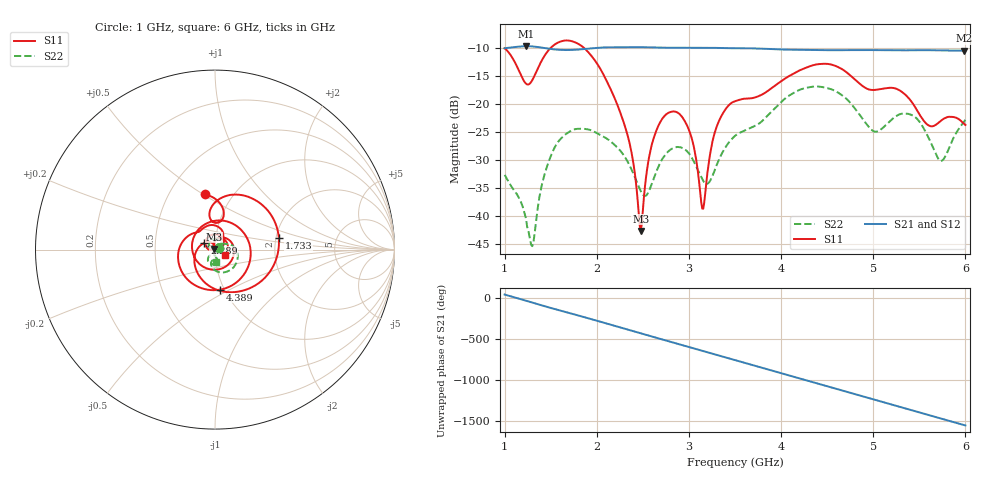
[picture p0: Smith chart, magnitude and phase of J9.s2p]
!Agilent Technologies,E8364B,MY43040528,A.07.50.67
!Agilent E8364B: A.07.50.67
!Date: Sunday, March 01, 2026 19:10:28
!Correction: S11(Full 2 Port(1,2))
!S21(Full 2 Port(1,2))
!S12(Full 2 Port(1,2))
!S22(Full 2 Port(1,2))
!S2P File: Measurements: S11, S21, S12, S22:
# Hz S  dB  R 50
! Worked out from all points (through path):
!   451 points, 1 GHz to 6 GHz, reference 50 ohm
!   highest |S21| = -9.72 dB at 1.233 GHz (marker M1); lowest = -10.5 dB at 5.989 GHz (marker M2)
!   group delay of S21, straight-line fit = 889 ps
!   lowest |S11| = -42.6 dB at 2.478 GHz (marker M3), VSWR 1.01, Z = 49.4 + j0.414 ohm
!   |S11| at or under -10 dB: start of sweep to 1.501 GHz; 1.86 GHz to end of sweep
!   |S22| runs from -45.4 to -16.9 dB; largest |S21 - S12| = 0.0014
!   S11 on the Smith chart (normalised r, x): 1 GHz: 0.74, +0.51; 1.733 GHz: 2.08, +0.30; 2.289 GHz: 0.89, +0.07; 4.389 GHz: 0.95, -0.45; 6 GHz: 1.12, -0.06
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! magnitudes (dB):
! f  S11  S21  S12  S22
! 1 GHz  -10.1  -10.1  -10.1  -32.7
! 1.233 GHz  -16.4  -9.7  -9.8  -40.5
! 1.3 GHz  -15.8  -9.8  -9.8  -45.4
! 1.478 GHz  -10.4  -10.2  -10.2  -30.3
! 1.733 GHz  -8.8  -10.4  -10.4  -24.7
! 1.844 GHz  -9.8  -10.3  -10.3  -24.4
! 2.289 GHz  -23.1  -9.9  -9.9  -29.0
! 2.478 GHz  -42.6  -9.9  -9.9  -35.5
! 2.567 GHz  -29.6  -9.9  -10.0  -35.5
! 2.667 GHz  -24.0  -10.0  -10.0  -31.3
! 2.956 GHz  -23.1  -10.0  -10.0  -28.1
! 3.156 GHz  -38.7  -10.0  -10.0  -33.7
! 3.289 GHz  -24.6  -10.0  -10.0  -31.4
! 3.5 GHz  -19.5  -10.1  -10.1  -25.7
! 4.344 GHz  -13.1  -10.4  -10.4  -16.9
! 4.389 GHz  -13.0  -10.4  -10.4  -16.9
! 5 GHz  -17.5  -10.4  -10.4  -24.8
! 5.167 GHz  -17.1  -10.4  -10.5  -23.3
! 5.444 GHz  -20.3  -10.4  -10.5  -22.2
! 5.733 GHz  -23.0  -10.5  -10.5  -30.2
! 5.989 GHz  -23.6  -10.5  -10.5  -23.1
! 6 GHz  -23.8  -10.5  -10.5  -22.8
